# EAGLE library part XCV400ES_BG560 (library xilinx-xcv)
xcv400es_bg560 edit this description Auto generated by make-symbol-device-package-bsdl.ulp Rev. 26 Source: xcv400es_bg560.bsd
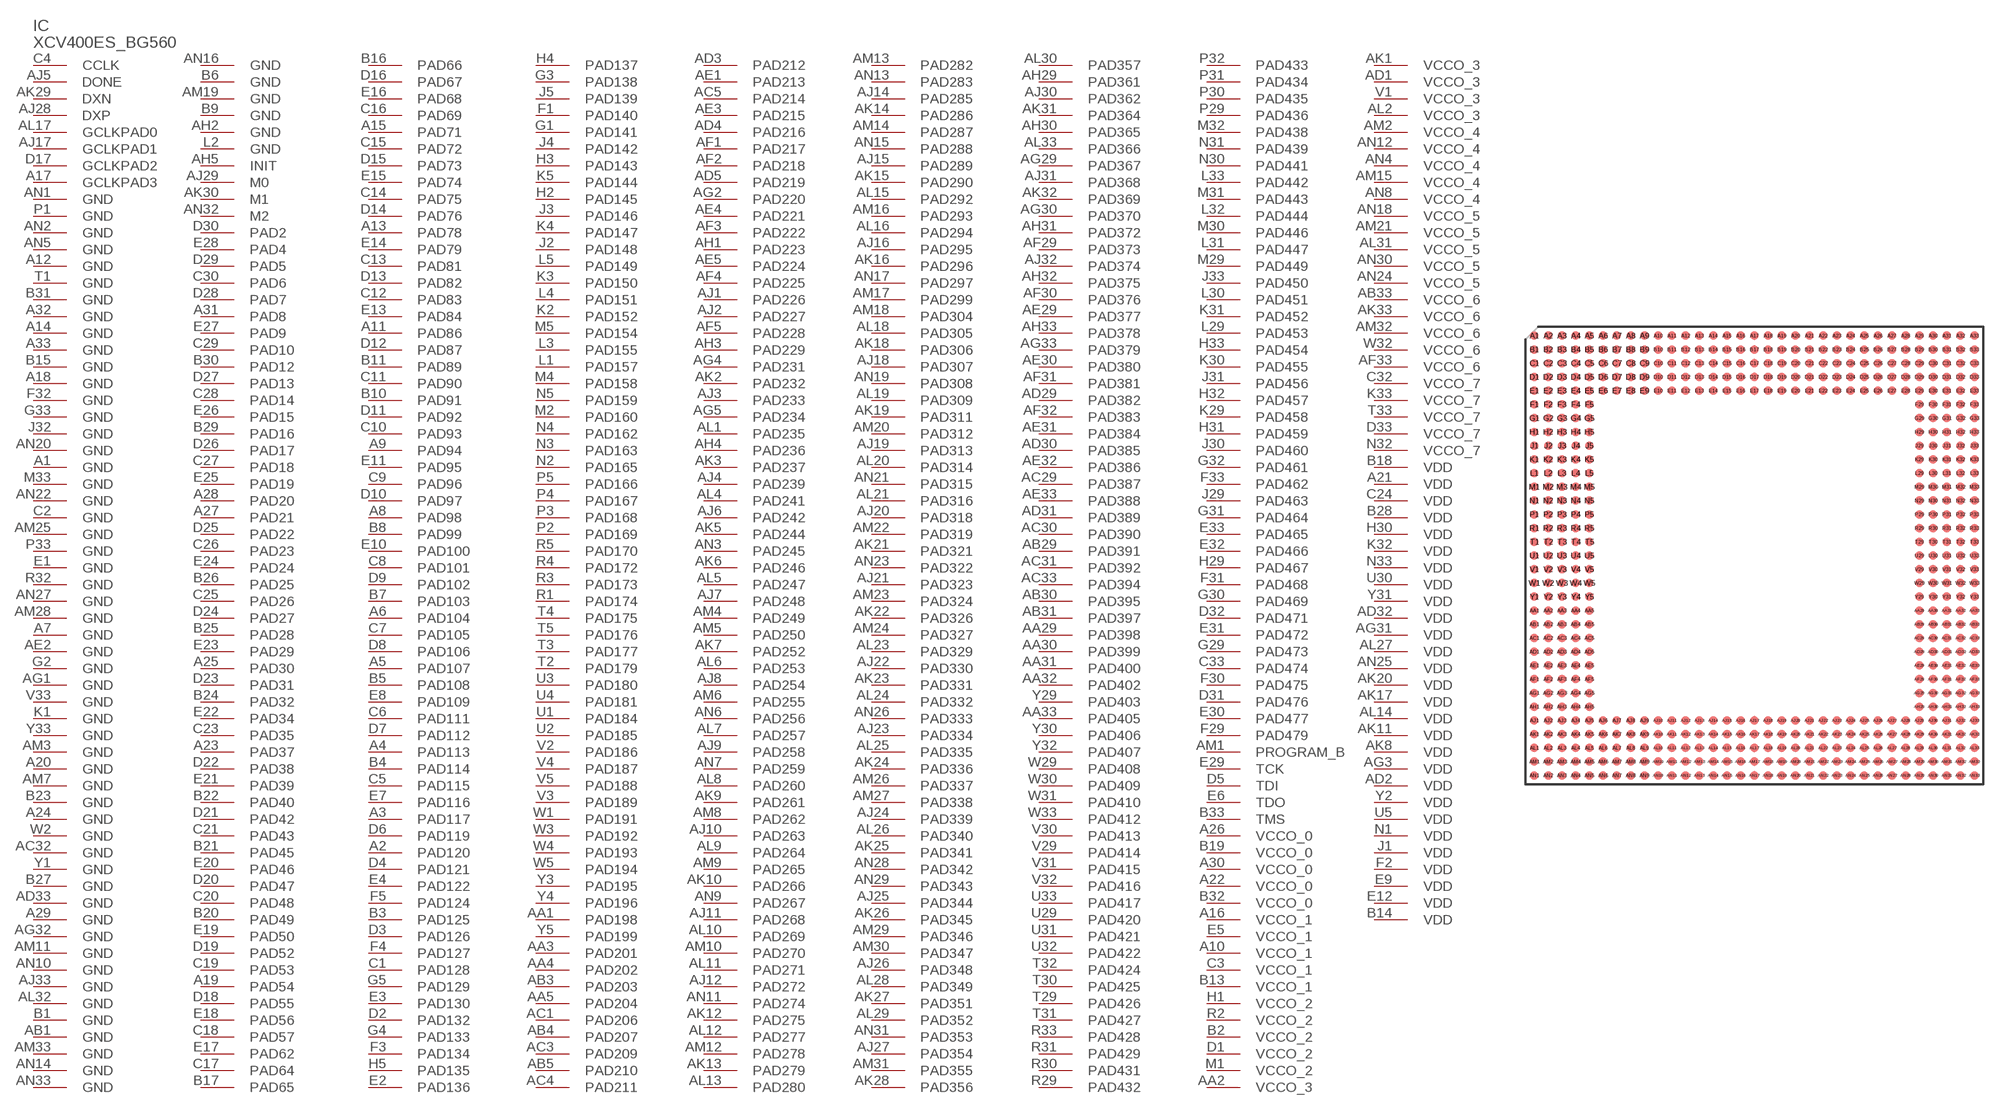
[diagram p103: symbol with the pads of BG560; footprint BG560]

Designator prefix IC

## XCV400ES_BG560 (OC_FARNELL: unknown; OC_NEWARK: unknown)  [BG560]
A1  GND  pwr
A2  PAD120
A3  PAD117
A4  PAD113
A5  PAD107
A6  PAD104
A7  GND  pwr
A8  PAD98
A9  PAD94
A10  VCCO_1  pwr
A11  PAD86
A12  GND  pwr
A13  PAD78
A14  GND  pwr
A15  PAD71
A16  VCCO_1  pwr
A17  GCLKPAD3  in
A18  GND  pwr
A19  PAD54
A20  GND  pwr
A21  VDD  pwr
A22  VCCO_0  pwr
A23  PAD37
A24  GND  pwr
A25  PAD30
A26  VCCO_0  pwr
A27  PAD21
A28  PAD20
A29  GND  pwr
A30  VCCO_0  pwr
A31  PAD8
A32  GND  pwr
A33  GND  pwr
AA1  PAD198
AA2  VCCO_3  pwr
AA3  PAD201
AA4  PAD202
AA5  PAD204
AA29  PAD398
AA30  PAD399
AA31  PAD400
AA32  PAD402
AA33  PAD405
AB1  GND  pwr
AB3  PAD203
AB4  PAD207
AB5  PAD210
AB29  PAD391
AB30  PAD395
AB31  PAD397
AB33  VCCO_6  pwr
AC1  PAD206
AC3  PAD209
AC4  PAD211
AC5  PAD214
AC29  PAD387
AC30  PAD390
AC31  PAD392
AC32  GND  pwr
AC33  PAD394
AD1  VCCO_3  pwr
AD2  VDD  pwr
AD3  PAD212
AD4  PAD216
AD5  PAD219
AD29  PAD382
AD30  PAD385
AD31  PAD389
AD32  VDD  pwr
AD33  GND  pwr
AE1  PAD213
AE2  GND  pwr
AE3  PAD215
AE4  PAD221
AE5  PAD224
AE29  PAD377
AE30  PAD380
AE31  PAD384
AE32  PAD386
AE33  PAD388
AF1  PAD217
AF2  PAD218
AF3  PAD222
AF4  PAD225
AF5  PAD228
AF29  PAD373
AF30  PAD376
AF31  PAD381
AF32  PAD383
AF33  VCCO_6  pwr
AG1  GND  pwr
AG2  PAD220
AG3  VDD  pwr
AG4  PAD231
AG5  PAD234
AG29  PAD367
AG30  PAD370
AG31  VDD  pwr
AG32  GND  pwr
AG33  PAD379
AH1  PAD223
AH2  GND  pwr
AH3  PAD229
AH4  PAD236
AH5  INIT
AH29  PAD361
AH30  PAD365
AH31  PAD372
AH32  PAD375
AH33  PAD378
AJ1  PAD226
AJ2  PAD227
AJ3  PAD233
AJ4  PAD239
AJ5  DONE
AJ6  PAD242
AJ7  PAD248
AJ8  PAD254
AJ9  PAD258
AJ10  PAD263
AJ11  PAD268
AJ12  PAD272
AJ14  PAD285
AJ15  PAD289
AJ16  PAD295
AJ17  GCLKPAD1  in
AJ18  PAD307
AJ19  PAD313
AJ20  PAD318
AJ21  PAD323
AJ22  PAD330
AJ23  PAD334
AJ24  PAD339
AJ25  PAD344
AJ26  PAD348
AJ27  PAD354
AJ28  DXP  pas
AJ29  M0  in
AJ30  PAD362
AJ31  PAD368
AJ32  PAD374
AJ33  GND  pwr
AK1  VCCO_3  pwr
AK2  PAD232
AK3  PAD237
AK5  PAD244
AK6  PAD246
AK7  PAD252
AK8  VDD  pwr
AK9  PAD261
AK10  PAD266
AK11  VDD  pwr
AK12  PAD275
AK13  PAD279
AK14  PAD286
AK15  PAD290
AK16  PAD296
AK17  VDD  pwr
AK18  PAD306
AK19  PAD311
AK20  VDD  pwr
AK21  PAD321
AK22  PAD326
AK23  PAD331
AK24  PAD336
AK25  PAD341
AK26  PAD345
AK27  PAD351
AK28  PAD356
AK29  DXN  pas
AK30  M1  in
AK31  PAD364
AK32  PAD369
AK33  VCCO_6  pwr
AL1  PAD235
AL2  VCCO_3  pwr
AL4  PAD241
AL5  PAD247
AL6  PAD253
AL7  PAD257
AL8  PAD260
AL9  PAD264
AL10  PAD269
AL11  PAD271
AL12  PAD277
AL13  PAD280
AL14  VDD  pwr
AL15  PAD292
AL16  PAD294
AL17  GCLKPAD0  in
AL18  PAD305
AL19  PAD309
AL20  PAD314
AL21  PAD316
AL23  PAD329
AL24  PAD332
AL25  PAD335
AL26  PAD340
AL27  VDD  pwr
AL28  PAD349
AL29  PAD352
AL30  PAD357
AL31  VCCO_5  pwr
AL32  GND  pwr
AL33  PAD366
AM1  PROGRAM_B  in
AM2  VCCO_4  pwr
AM3  GND  pwr
AM4  PAD249
AM5  PAD250
AM6  PAD255
AM7  GND  pwr
AM8  PAD262
AM9  PAD265
AM10  PAD270
AM11  GND  pwr
AM12  PAD278
AM13  PAD282
AM14  PAD287
AM15  VCCO_4  pwr
AM16  PAD293
AM17  PAD299
AM18  PAD304
AM19  GND  pwr
AM20  PAD312
AM21  VCCO_5  pwr
AM22  PAD319
AM23  PAD324
AM24  PAD327
AM25  GND  pwr
AM26  PAD337
AM27  PAD338
AM28  GND  pwr
AM29  PAD346
AM30  PAD347
AM31  PAD355
AM32  VCCO_6  pwr
AM33  GND  pwr
AN1  GND  pwr
AN2  GND  pwr
AN3  PAD245
AN4  VCCO_4  pwr
AN5  GND  pwr
AN6  PAD256
AN7  PAD259
AN8  VCCO_4  pwr
AN9  PAD267
AN10  GND  pwr
AN11  PAD274
AN12  VCCO_4  pwr
AN13  PAD283
AN14  GND  pwr
AN15  PAD288
AN16  GND  pwr
AN17  PAD297
AN18  VCCO_5  pwr
AN19  PAD308
AN20  GND  pwr
AN21  PAD315
AN22  GND  pwr
AN23  PAD322
AN24  VCCO_5  pwr
AN25  VDD  pwr
AN26  PAD333
AN27  GND  pwr
AN28  PAD342
AN29  PAD343
AN30  VCCO_5  pwr
AN31  PAD353
AN32  M2  in
AN33  GND  pwr
B1  GND  pwr
B2  VCCO_2  pwr
B3  PAD125
B4  PAD114
B5  PAD108
B6  GND  pwr
B7  PAD103
B8  PAD99
B9  GND  pwr
B10  PAD91
B11  PAD89
B13  VCCO_1  pwr
B14  VDD  pwr
B15  GND  pwr
B16  PAD66
B17  PAD65
B18  VDD  pwr
B19  VCCO_0  pwr
B20  PAD49
B21  PAD45
B22  PAD40
B23  GND  pwr
B24  PAD32
B25  PAD28
B26  PAD25
B27  GND  pwr
B28  VDD  pwr
B29  PAD16
B30  PAD12
B31  GND  pwr
B32  VCCO_0  pwr
B33  TMS  in
C1  PAD128
C2  GND  pwr
C3  VCCO_1  pwr
C4  CCLK
C5  PAD115
C6  PAD111
C7  PAD105
C8  PAD101
C9  PAD96
C10  PAD93
C11  PAD90
C12  PAD83
C13  PAD81
C14  PAD75
C15  PAD72
C16  PAD69
C17  PAD64
C18  PAD57
C19  PAD53
C20  PAD48
C21  PAD43
C23  PAD35
C24  VDD  pwr
C25  PAD26
C26  PAD23
C27  PAD18
C28  PAD14
C29  PAD10
C30  PAD6
C32  VCCO_7  pwr
C33  PAD474
D1  VCCO_2  pwr
D2  PAD132
D3  PAD126
D4  PAD121
D5  TDI  in
D6  PAD119
D7  PAD112
D8  PAD106
D9  PAD102
D10  PAD97
D11  PAD92
D12  PAD87
D13  PAD82
D14  PAD76
D15  PAD73
D16  PAD67
D17  GCLKPAD2  in
D18  PAD55
D19  PAD52
D20  PAD47
D21  PAD42
D22  PAD38
D23  PAD31
D24  PAD27
D25  PAD22
D26  PAD17
D27  PAD13
D28  PAD7
D29  PAD5
D30  PAD2
D31  PAD476
D32  PAD471
D33  VCCO_7  pwr
E1  GND  pwr
E2  PAD136
E3  PAD130
E4  PAD122
E5  VCCO_1  pwr
E6  TDO  out
E7  PAD116
E8  PAD109
E9  VDD  pwr
E10  PAD100
E11  PAD95
E12  VDD  pwr
E13  PAD84
E14  PAD79
E15  PAD74
E16  PAD68
E17  PAD62
E18  PAD56
E19  PAD50
E20  PAD46
E21  PAD39
E22  PAD34
E23  PAD29
E24  PAD24
E25  PAD19
E26  PAD15
E27  PAD9
E28  PAD4
E29  TCK  in
E30  PAD477
E31  PAD472
E32  PAD466
E33  PAD465
F1  PAD140
F2  VDD  pwr
F3  PAD134
F4  PAD127
F5  PAD124
F29  PAD479
F30  PAD475
F31  PAD468
F32  GND  pwr
F33  PAD462
G1  PAD141
G2  GND  pwr
G3  PAD138
G4  PAD133
G5  PAD129
G29  PAD473
G30  PAD469
G31  PAD464
G32  PAD461
G33  GND  pwr
H1  VCCO_2  pwr
H2  PAD145
H3  PAD143
H4  PAD137
H5  PAD135
H29  PAD467
H30  VDD  pwr
H31  PAD459
H32  PAD457
H33  PAD454
J1  VDD  pwr
J2  PAD148
J3  PAD146
J4  PAD142
J5  PAD139
J29  PAD463
J30  PAD460
J31  PAD456
J32  GND  pwr
J33  PAD450
K1  GND  pwr
K2  PAD152
K3  PAD150
K4  PAD147
K5  PAD144
K29  PAD458
K30  PAD455
K31  PAD452
K32  VDD  pwr
K33  VCCO_7  pwr
L1  PAD157
L2  GND  pwr
L3  PAD155
L4  PAD151
L5  PAD149
L29  PAD453
L30  PAD451
L31  PAD447
L32  PAD444
L33  PAD442
M1  VCCO_2  pwr
M2  PAD160
M4  PAD158
M5  PAD154
M29  PAD449
M30  PAD446
M31  PAD443
M32  PAD438
M33  GND  pwr
N1  VDD  pwr
N2  PAD165
N3  PAD163
N4  PAD162
N5  PAD159
N30  PAD441
N31  PAD439
N32  VCCO_7  pwr
N33  VDD  pwr
P1  GND  pwr
P2  PAD169
P3  PAD168
P4  PAD167
P5  PAD166
P29  PAD436
P30  PAD435
P31  PAD434
P32  PAD433
P33  GND  pwr
R1  PAD174
R2  VCCO_2  pwr
R3  PAD173
R4  PAD172
R5  PAD170
R29  PAD432
R30  PAD431
R31  PAD429
R32  GND  pwr
R33  PAD428
T1  GND  pwr
T2  PAD179
T3  PAD177
T4  PAD175
T5  PAD176
T29  PAD426
T30  PAD425
T31  PAD427
T32  PAD424
T33  VCCO_7  pwr
U1  PAD184
U2  PAD185
U3  PAD180
U4  PAD181
U5  VDD  pwr
U29  PAD420
U30  VDD  pwr
U31  PAD421
U32  PAD422
U33  PAD417
V1  VCCO_3  pwr
V2  PAD186
V3  PAD189
V4  PAD187
V5  PAD188
V29  PAD414
V30  PAD413
V31  PAD415
V32  PAD416
V33  GND  pwr
W1  PAD191
W2  GND  pwr
W3  PAD192
W4  PAD193
W5  PAD194
W29  PAD408
W30  PAD409
W31  PAD410
W32  VCCO_6  pwr
W33  PAD412
Y1  GND  pwr
Y2  VDD  pwr
Y3  PAD195
Y4  PAD196
Y5  PAD199
Y29  PAD403
Y30  PAD406
Y31  VDD  pwr
Y32  PAD407
Y33  GND  pwr

## Footprint BG560 (pad centres in mm)
Metal BGA (BG560) Auto generated by make-symbol-device-package-bsdl.ulp Rev. 26 Source: xcv1000_bg560_1532.bsd; bg560.pdf
smd 0.8 x 0.8: A1 -20.32,20.32; A2 -19.05,20.32; A3 -17.78,20.32; A4 -16.51,20.32; A5 -15.24,20.32; A6 -13.97,20.32; A7 -12.7,20.32; A8 -11.43,20.32; A9 -10.16,20.32; A10 -8.89,20.32; A11 -7.62,20.32; A12 -6.35,20.32; A13 -5.08,20.32; A14 -3.81,20.32; A15 -2.54,20.32; A16 -1.27,20.32; A17 0,20.32; A18 1.27,20.32; A19 2.54,20.32; A20 3.81,20.32; A21 5.08,20.32; A22 6.35,20.32; A23 7.62,20.32; A24 8.89,20.32; A25 10.16,20.32; A26 11.43,20.32; A27 12.7,20.32; A28 13.97,20.32; A29 15.24,20.32; A30 16.51,20.32; A31 17.78,20.32; A32 19.05,20.32; A33 20.32,20.32; AA1 -20.32,-5.08; AA2 -19.05,-5.08; AA3 -17.78,-5.08; AA4 -16.51,-5.08; AA5 -15.24,-5.08; AA29 15.24,-5.08; AA30 16.51,-5.08; AA31 17.78,-5.08; AA32 19.05,-5.08; AA33 20.32,-5.08; AB1 -20.32,-6.35; AB2 -19.05,-6.35; AB3 -17.78,-6.35; AB4 -16.51,-6.35; AB5 -15.24,-6.35; AB29 15.24,-6.35; AB30 16.51,-6.35; AB31 17.78,-6.35; AB32 19.05,-6.35; AB33 20.32,-6.35; AC1 -20.32,-7.62; AC2 -19.05,-7.62; AC3 -17.78,-7.62; AC4 -16.51,-7.62; AC5 -15.24,-7.62; AC29 15.24,-7.62; AC30 16.51,-7.62; AC31 17.78,-7.62; AC32 19.05,-7.62; AC33 20.32,-7.62; AD1 -20.32,-8.89; AD2 -19.05,-8.89; AD3 -17.78,-8.89; AD4 -16.51,-8.89; AD5 -15.24,-8.89; AD29 15.24,-8.89; AD30 16.51,-8.89; AD31 17.78,-8.89; AD32 19.05,-8.89; AD33 20.32,-8.89; AE1 -20.32,-10.16; AE2 -19.05,-10.16; AE3 -17.78,-10.16; AE4 -16.51,-10.16; AE5 -15.24,-10.16; AE29 15.24,-10.16; AE30 16.51,-10.16; AE31 17.78,-10.16; AE32 19.05,-10.16; AE33 20.32,-10.16; AF1 -20.32,-11.43; AF2 -19.05,-11.43; AF3 -17.78,-11.43; AF4 -16.51,-11.43; AF5 -15.24,-11.43; AF29 15.24,-11.43; AF30 16.51,-11.43; AF31 17.78,-11.43; AF32 19.05,-11.43; AF33 20.32,-11.43; AG1 -20.32,-12.7; AG2 -19.05,-12.7; AG3 -17.78,-12.7; AG4 -16.51,-12.7; AG5 -15.24,-12.7; AG29 15.24,-12.7; AG30 16.51,-12.7; AG31 17.78,-12.7; AG32 19.05,-12.7; AG33 20.32,-12.7; AH1 -20.32,-13.97; AH2 -19.05,-13.97; AH3 -17.78,-13.97; AH4 -16.51,-13.97; AH5 -15.24,-13.97; AH29 15.24,-13.97; AH30 16.51,-13.97; AH31 17.78,-13.97; AH32 19.05,-13.97; AH33 20.32,-13.97; AJ1 -20.32,-15.24; AJ2 -19.05,-15.24; AJ3 -17.78,-15.24; AJ4 -16.51,-15.24; AJ5 -15.24,-15.24; AJ6 -13.97,-15.24; AJ7 -12.7,-15.24; AJ8 -11.43,-15.24; AJ9 -10.16,-15.24; AJ10 -8.89,-15.24; AJ11 -7.62,-15.24; AJ12 -6.35,-15.24; AJ13 -5.08,-15.24; AJ14 -3.81,-15.24; AJ15 -2.54,-15.24; AJ16 -1.27,-15.24; AJ17 0,-15.24; AJ18 1.27,-15.24; AJ19 2.54,-15.24; AJ20 3.81,-15.24; AJ21 5.08,-15.24; AJ22 6.35,-15.24; AJ23 7.62,-15.24; AJ24 8.89,-15.24; AJ25 10.16,-15.24; AJ26 11.43,-15.24; AJ27 12.7,-15.24; AJ28 13.97,-15.24; AJ29 15.24,-15.24; AJ30 16.51,-15.24; AJ31 17.78,-15.24; AJ32 19.05,-15.24; AJ33 20.32,-15.24; AK1 -20.32,-16.51; AK2 -19.05,-16.51; AK3 -17.78,-16.51; AK4 -16.51,-16.51; AK5 -15.24,-16.51; AK6 -13.97,-16.51; AK7 -12.7,-16.51; AK8 -11.43,-16.51; AK9 -10.16,-16.51; AK10 -8.89,-16.51; AK11 -7.62,-16.51; AK12 -6.35,-16.51; AK13 -5.08,-16.51; AK14 -3.81,-16.51; AK15 -2.54,-16.51; AK16 -1.27,-16.51; AK17 0,-16.51; AK18 1.27,-16.51; AK19 2.54,-16.51; AK20 3.81,-16.51; AK21 5.08,-16.51; AK22 6.35,-16.51; AK23 7.62,-16.51; AK24 8.89,-16.51; AK25 10.16,-16.51; AK26 11.43,-16.51; AK27 12.7,-16.51; AK28 13.97,-16.51; AK29 15.24,-16.51; AK30 16.51,-16.51; AK31 17.78,-16.51; AK32 19.05,-16.51; AK33 20.32,-16.51; AL1 -20.32,-17.78; AL2 -19.05,-17.78; AL3 -17.78,-17.78; AL4 -16.51,-17.78; AL5 -15.24,-17.78; AL6 -13.97,-17.78; AL7 -12.7,-17.78; AL8 -11.43,-17.78; AL9 -10.16,-17.78; AL10 -8.89,-17.78; AL11 -7.62,-17.78; AL12 -6.35,-17.78; AL13 -5.08,-17.78; AL14 -3.81,-17.78; AL15 -2.54,-17.78; AL16 -1.27,-17.78; AL17 0,-17.78; AL18 1.27,-17.78; AL19 2.54,-17.78; AL20 3.81,-17.78; AL21 5.08,-17.78; AL22 6.35,-17.78; AL23 7.62,-17.78; AL24 8.89,-17.78; AL25 10.16,-17.78; AL26 11.43,-17.78; AL27 12.7,-17.78; AL28 13.97,-17.78; AL29 15.24,-17.78; AL30 16.51,-17.78; AL31 17.78,-17.78; AL32 19.05,-17.78; AL33 20.32,-17.78; AM1 -20.32,-19.05; AM2 -19.05,-19.05; AM3 -17.78,-19.05; AM4 -16.51,-19.05; AM5 -15.24,-19.05; AM6 -13.97,-19.05; AM7 -12.7,-19.05; AM8 -11.43,-19.05; AM9 -10.16,-19.05; AM10 -8.89,-19.05; AM11 -7.62,-19.05; AM12 -6.35,-19.05; AM13 -5.08,-19.05; AM14 -3.81,-19.05; AM15 -2.54,-19.05; AM16 -1.27,-19.05; AM17 0,-19.05; AM18 1.27,-19.05; AM19 2.54,-19.05; AM20 3.81,-19.05; AM21 5.08,-19.05; AM22 6.35,-19.05; AM23 7.62,-19.05; AM24 8.89,-19.05; AM25 10.16,-19.05; AM26 11.43,-19.05; AM27 12.7,-19.05; AM28 13.97,-19.05; AM29 15.24,-19.05; AM30 16.51,-19.05; AM31 17.78,-19.05; AM32 19.05,-19.05; AM33 20.32,-19.05; AN1 -20.32,-20.32; AN2 -19.05,-20.32; AN3 -17.78,-20.32; AN4 -16.51,-20.32; AN5 -15.24,-20.32; AN6 -13.97,-20.32; AN7 -12.7,-20.32; AN8 -11.43,-20.32; AN9 -10.16,-20.32; AN10 -8.89,-20.32; AN11 -7.62,-20.32; AN12 -6.35,-20.32; AN13 -5.08,-20.32; AN14 -3.81,-20.32; AN15 -2.54,-20.32; AN16 -1.27,-20.32; AN17 0,-20.32; AN18 1.27,-20.32; AN19 2.54,-20.32; AN20 3.81,-20.32; AN21 5.08,-20.32; AN22 6.35,-20.32; AN23 7.62,-20.32; AN24 8.89,-20.32; AN25 10.16,-20.32; AN26 11.43,-20.32; AN27 12.7,-20.32; AN28 13.97,-20.32; AN29 15.24,-20.32; AN30 16.51,-20.32; AN31 17.78,-20.32; AN32 19.05,-20.32; AN33 20.32,-20.32; B1 -20.32,19.05; B2 -19.05,19.05; B3 -17.78,19.05; B4 -16.51,19.05; B5 -15.24,19.05; B6 -13.97,19.05; B7 -12.7,19.05; B8 -11.43,19.05; B9 -10.16,19.05; B10 -8.89,19.05; B11 -7.62,19.05; B12 -6.35,19.05; B13 -5.08,19.05; B14 -3.81,19.05; B15 -2.54,19.05; B16 -1.27,19.05; B17 0,19.05; B18 1.27,19.05; B19 2.54,19.05; B20 3.81,19.05; B21 5.08,19.05; B22 6.35,19.05; B23 7.62,19.05; B24 8.89,19.05; B25 10.16,19.05; B26 11.43,19.05; B27 12.7,19.05; B28 13.97,19.05; B29 15.24,19.05; B30 16.51,19.05; B31 17.78,19.05; B32 19.05,19.05; B33 20.32,19.05; C1 -20.32,17.78; C2 -19.05,17.78; C3 -17.78,17.78; C4 -16.51,17.78; C5 -15.24,17.78; C6 -13.97,17.78; C7 -12.7,17.78; C8 -11.43,17.78; C9 -10.16,17.78; C10 -8.89,17.78; C11 -7.62,17.78; C12 -6.35,17.78; C13 -5.08,17.78; C14 -3.81,17.78; C15 -2.54,17.78; C16 -1.27,17.78; C17 0,17.78; C18 1.27,17.78; C19 2.54,17.78; C20 3.81,17.78; C21 5.08,17.78; C22 6.35,17.78; C23 7.62,17.78; C24 8.89,17.78; C25 10.16,17.78; C26 11.43,17.78; C27 12.7,17.78; C28 13.97,17.78; C29 15.24,17.78; C30 16.51,17.78; C31 17.78,17.78; C32 19.05,17.78; C33 20.32,17.78; D1 -20.32,16.51; D2 -19.05,16.51; D3 -17.78,16.51; D4 -16.51,16.51; D5 -15.24,16.51; D6 -13.97,16.51; D7 -12.7,16.51; D8 -11.43,16.51; D9 -10.16,16.51; D10 -8.89,16.51; D11 -7.62,16.51; D12 -6.35,16.51; D13 -5.08,16.51; D14 -3.81,16.51; D15 -2.54,16.51; D16 -1.27,16.51; D17 0,16.51; D18 1.27,16.51; D19 2.54,16.51; D20 3.81,16.51; D21 5.08,16.51; D22 6.35,16.51; D23 7.62,16.51; D24 8.89,16.51; D25 10.16,16.51; D26 11.43,16.51; D27 12.7,16.51; D28 13.97,16.51; D29 15.24,16.51; D30 16.51,16.51; D31 17.78,16.51; D32 19.05,16.51; D33 20.32,16.51; E1 -20.32,15.24; E2 -19.05,15.24; E3 -17.78,15.24; E4 -16.51,15.24; E5 -15.24,15.24; E6 -13.97,15.24; E7 -12.7,15.24; E8 -11.43,15.24; E9 -10.16,15.24; E10 -8.89,15.24; E11 -7.62,15.24; E12 -6.35,15.24; E13 -5.08,15.24; E14 -3.81,15.24; E15 -2.54,15.24; E16 -1.27,15.24; E17 0,15.24; E18 1.27,15.24; E19 2.54,15.24; E20 3.81,15.24; E21 5.08,15.24; E22 6.35,15.24; E23 7.62,15.24; E24 8.89,15.24; E25 10.16,15.24; E26 11.43,15.24; E27 12.7,15.24; E28 13.97,15.24; E29 15.24,15.24; E30 16.51,15.24; E31 17.78,15.24; E32 19.05,15.24; E33 20.32,15.24; F1 -20.32,13.97; F2 -19.05,13.97; F3 -17.78,13.97; F4 -16.51,13.97; F5 -15.24,13.97; F29 15.24,13.97; F30 16.51,13.97; F31 17.78,13.97; F32 19.05,13.97; F33 20.32,13.97; G1 -20.32,12.7; G2 -19.05,12.7; G3 -17.78,12.7; G4 -16.51,12.7; G5 -15.24,12.7; G29 15.24,12.7; G30 16.51,12.7; G31 17.78,12.7; G32 19.05,12.7; G33 20.32,12.7; H1 -20.32,11.43; H2 -19.05,11.43; H3 -17.78,11.43; H4 -16.51,11.43; H5 -15.24,11.43; H29 15.24,11.43; H30 16.51,11.43; H31 17.78,11.43; H32 19.05,11.43; H33 20.32,11.43; J1 -20.32,10.16; J2 -19.05,10.16; J3 -17.78,10.16; J4 -16.51,10.16; J5 -15.24,10.16; J29 15.24,10.16; J30 16.51,10.16; J31 17.78,10.16; J32 19.05,10.16; J33 20.32,10.16; K1 -20.32,8.89; K2 -19.05,8.89; K3 -17.78,8.89; K4 -16.51,8.89; K5 -15.24,8.89; K29 15.24,8.89; K30 16.51,8.89; K31 17.78,8.89; K32 19.05,8.89; K33 20.32,8.89; L1 -20.32,7.62; L2 -19.05,7.62; L3 -17.78,7.62; L4 -16.51,7.62; L5 -15.24,7.62; L29 15.24,7.62; L30 16.51,7.62; L31 17.78,7.62; L32 19.05,7.62; L33 20.32,7.62; M1 -20.32,6.35; M2 -19.05,6.35; M3 -17.78,6.35; M4 -16.51,6.35; M5 -15.24,6.35; M29 15.24,6.35; M30 16.51,6.35; M31 17.78,6.35; M32 19.05,6.35; M33 20.32,6.35; N1 -20.32,5.08; N2 -19.05,5.08; N3 -17.78,5.08; N4 -16.51,5.08; N5 -15.24,5.08; N29 15.24,5.08; N30 16.51,5.08; N31 17.78,5.08; N32 19.05,5.08; N33 20.32,5.08; P1 -20.32,3.81; P2 -19.05,3.81; P3 -17.78,3.81; P4 -16.51,3.81; P5 -15.24,3.81; P29 15.24,3.81; P30 16.51,3.81; P31 17.78,3.81; P32 19.05,3.81; P33 20.32,3.81; R1 -20.32,2.54; R2 -19.05,2.54; R3 -17.78,2.54; R4 -16.51,2.54; R5 -15.24,2.54; R29 15.24,2.54; R30 16.51,2.54; R31 17.78,2.54; R32 19.05,2.54; R33 20.32,2.54; T1 -20.32,1.27; T2 -19.05,1.27; T3 -17.78,1.27; T4 -16.51,1.27; T5 -15.24,1.27; T29 15.24,1.27; T30 16.51,1.27; T31 17.78,1.27; T32 19.05,1.27; T33 20.32,1.27; U1 -20.32,0; U2 -19.05,0; U3 -17.78,0; U4 -16.51,0; U5 -15.24,0; U29 15.24,0; U30 16.51,0; U31 17.78,0; U32 19.05,0; U33 20.32,0; V1 -20.32,-1.27; V2 -19.05,-1.27; V3 -17.78,-1.27; V4 -16.51,-1.27; V5 -15.24,-1.27; V29 15.24,-1.27; V30 16.51,-1.27; V31 17.78,-1.27; V32 19.05,-1.27; V33 20.32,-1.27; W1 -20.32,-2.54; W2 -19.05,-2.54; W3 -17.78,-2.54; W4 -16.51,-2.54; W5 -15.24,-2.54; W29 15.24,-2.54; W30 16.51,-2.54; W31 17.78,-2.54; W32 19.05,-2.54; W33 20.32,-2.54; Y1 -20.32,-3.81; Y2 -19.05,-3.81; Y3 -17.78,-3.81; Y4 -16.51,-3.81; Y5 -15.24,-3.81; Y29 15.24,-3.81; Y30 16.51,-3.81; Y31 17.78,-3.81; Y32 19.05,-3.81; Y33 20.32,-3.81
